// TwinCAT 3 PLC project UPS_IPC_test
// ProgramVersion: 3.1.4023.0
// libraries:
//   Tc2_Standard, * (Beckhoff Automation GmbH)
//   Tc2_System, * (Beckhoff Automation GmbH)
//   Tc2_Utilities, * (Beckhoff Automation GmbH)
//   Tc3_Module, * (Beckhoff Automation GmbH)
// project tree:
//   / PlcTask.TcTTO
//   POUs/ MAIN.TcPOU
// real-time tasks:
//   TASK PlcTask: cycle T#10ms, priority 20, ADS port 350

CONFIGURATION UPS_IPC_test
    RESOURCE PLC ON TwinCAT3
        TASK PlcTask(INTERVAL := T#10ms, PRIORITY := 20);
        PROGRAM MAIN WITH PlcTask : MAIN;
    END_RESOURCE
END_CONFIGURATION

// ---- POUs/MAIN.TcPOU
PROGRAM MAIN
VAR
	b_pfail AT %I*: BOOL;								//用于接收CU8130-0120的P FAIL口输出的关闭Uin的输入电压
	b_upsen AT %Q*: BOOL:= TRUE;						//用于给CU8130-0120的UPS EN	口输入高电平，当P Fail口有输出时给UPS EN口一个下降沿用于关闭U1,2out的输出
	b_upsready AT %I*:BOOL;
	FB_WritePersistentData: FB_WritePersistentData;		//该功能块用于写入持续的数据起到掉电数据保存的功能
	b_start: BOOL;
	b_busy: BOOL;
	FB_TON: TON;
	b_PSHDN AT %Q*: BOOL;
END_VAR
VAR PERSISTENT
	Array_persistent: ARRAY[0..1048575] OF byte;
END_VAR

FB_WritePersistentData(
	NETID:= , 
	PORT:= 852, 
	START:= b_start, 
	TMOUT:= , 
	MODE:= , 
	BUSY=> b_busy, 
	ERR=> , 
	ERRID=> );
FB_TON(IN:= , PT:= T#15S, Q=> , ET=> );
IF b_pfail=TRUE THEN
	b_start:=TRUE;
	IF NOT(b_busy=TRUE) THEN
		FB_TON.IN:=TRUE;
		IF FB_TON.Q=TRUE THEN
			b_upsen:=FALSE;
		END_IF
	END_IF
ELSE b_upsen:=TRUE;
END_IF

END_PROGRAM
